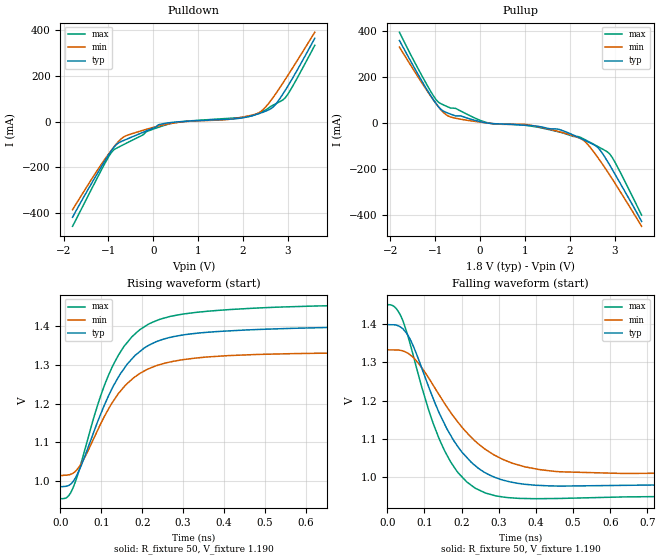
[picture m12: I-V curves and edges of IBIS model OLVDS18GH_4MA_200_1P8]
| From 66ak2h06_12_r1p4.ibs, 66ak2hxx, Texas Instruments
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[Model]   OLVDS18GH_4MA_200_1P8
Model_type   Output
Polarity   Non-Inverting
Cref =  15.0001pF
Rref =  101.0000M
Vref =  0V
Vmeas =  1.08V
C_comp   1p   1p   1p
[Temperature Range]   25   125   -40
[Voltage Range]   1.8   1.62   1.98
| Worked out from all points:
|   slope of the pulldown table from 0 to 0.27 V, typ, clamps not added: 12.8 ohm
|   slope of the pullup table from 0 to 0.27 V, typ, clamps not added: 32.8 ohm
|   rising waveform, R_fixture 50, V_fixture 1.190: 20-80 % time 114ps typ, 115ps min, 106ps max; typ from 0.986 V to 1.4 V
|   falling waveform, R_fixture 50, V_fixture 1.190: 20-80 % time 118ps typ, 152ps min, 102ps max; typ from 1.4 V to 0.985 V
| Nom Voltages:
[Pulldown]
|   voltage   I(typ)   I(min)   I(max)
-1.8V     -418.6mA   -385.5mA   -458.4mA
-1.091V   -175.8mA   -167.8mA   -187.3mA
-872.7mV  -110.9mA   -109.6mA   -122.6mA
-600mV    -77.61mA   -61.46mA   -94.58mA
-163.6mV  -41.62mA   -34.29mA   -45.1mA
163.6mV   -11.71mA   -17.18mA   -21.77mA
600mV     -528.8uA   -2.409mA   -1.429mA
1.691V    10.59mA    9.831mA    14.35mA
2.345V    34.17mA    37.59mA    36.12mA
2.673V    63.6mA     106.1mA    72.05mA
2.945V    138mA      185.7mA    105mA
3.6V      364.5mA    390.9mA    333.8mA
[Pullup]
|   voltage   I(typ)   I(min)   I(max)
-1.8V     359.9mA    331.1mA    395.8mA
-1.145V   132.4mA    129.1mA    152.1mA
-981.8mV  84.08mA    83.52mA    101.1mA
-872.7mV  58.82mA    56.76mA    83.68mA
-654.5mV  38.05mA    25.79mA    64.73mA
163.6mV   -565.4uA   -351.9uA   870.1uA
1.036V    -10.38mA   -7.223mA   -11.18mA
1.745V    -27.37mA   -37.12mA   -38.79mA
2.291V    -72.41mA   -74.36mA   -68.4mA
2.618V    -106.4mA   -149.9mA   -102.5mA
2.891V    -185.1mA   -228.4mA   -136.1mA
3.6V      -430.3mA   -451.5mA   -402.9mA
[Ramp]
| variable   typ   min   max
dV/dt_f   11.694m/1.0902515n   5.124m/0.87487225n   5.508m/0.60297483n
dV/dt_r   5.802m/0.89598732n   5.394m/3.4068839n   4.956m/0.56493914n
R_load = 50
[Rising Waveform]
R_fixture = 50
V_fixture = 1.190
V_fixture_min = 1.1743
V_fixture_max = 1.20176
|   time   V(typ)   V(min)   V(max)
0s        985.5mV    1.014V     954.5mV
18.9ps    988.1mV    1.016V     960.7mV
31.3ps    999.4mV    1.021V     983.6mV
52.7ps    1.045V     1.048V     1.054V
97.4ps    1.171V     1.146V     1.217V
139.9ps   1.265V     1.224V     1.322V
181.6ps   1.324V     1.269V     1.379V
241.2ps   1.363V     1.3V       1.417V
572.3ps   1.395V     1.329V     1.451V
1.312ns   1.399V     1.333V     1.452V
[Falling Waveform]
R_fixture = 50
V_fixture = 1.190
V_fixture_min = 1.1743
V_fixture_max = 1.20176
|   time   V(typ)   V(min)   V(max)
0s        1.399V     1.333V     1.451V
29.8ps    1.396V     1.332V     1.433V
55.5ps    1.371V     1.324V     1.369V
105.7ps   1.25V      1.268V     1.192V
155.1ps   1.137V     1.191V     1.067V
211ps     1.054V     1.119V     989.7mV
263.2ps   1.012V     1.073V     958.8mV
337.1ps   986.2mV    1.036V     945.6mV
465.2ps   976.6mV    1.014V     944.3mV
1.262ns   985.3mV    1.014V     954.4mV
